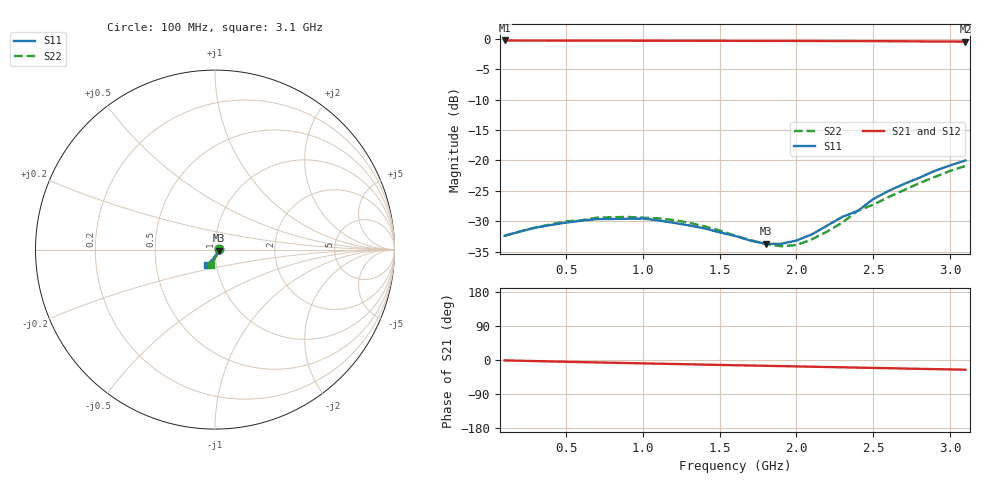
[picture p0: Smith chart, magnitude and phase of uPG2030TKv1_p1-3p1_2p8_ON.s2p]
! NEC Compound Semiconductor Devices Ltd.
! 21.January 2005
! uPG2030TK
! GaAs MMIC (0.1 - 3.1GHz SPDT switch)
! Vcont1=0v Vcont2=2.8v / IN-OUT1 ( ON )
! OUT2:50ohm termination
#  GHz  S  MA  R  50
!  f  S11  S21  S12  S22
!  GHz  MAG  ANG  MAG  ANG  MAG  ANG  MAG  ANG
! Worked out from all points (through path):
!   31 points, 100 MHz to 3.1 GHz, reference 50 ohm
!   highest |S21| = -0.25 dB at 100 MHz (marker M1); lowest = -0.4 dB at 3.1 GHz (marker M2)
!   group delay of S21, straight-line fit = 22.5 ps
!   lowest |S11| = -33.7 dB at 1.8 GHz (marker M3), VSWR 1.04, Z = 52 - j0.641 ohm
!   |S11| at or under -10 dB: start of sweep to end of sweep
!   |S22| runs from -34.1 to -20.9 dB; largest |S21 - S12| = 0.0034
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0.1  0.024 9.5  0.972 -1.0  0.971 -1.0  0.024 10.0
0.3  0.028 22.2  0.97 -2.9  0.97 -2.9  0.028 23.0
0.5  0.0308 28.7  0.969 -4.7  0.969 -4.7  0.0315 29.8
0.6  0.0319 32.3  0.9682 -5.6  0.9691 -5.6  0.0322 32.3
0.7  0.0329 32.0  0.9683 -6.4  0.9681 -6.4  0.0338 32.8
0.8  0.033 32.1  0.9677 -7.2  0.9676 -7.2  0.0341 33.7
1  0.0333 31.9  0.9672 -8.9  0.9665 -8.9  0.0338 34.4
1.1  0.0321 29.9  0.9666 -9.7  0.9667 -9.7  0.0334 32.8
1.3  0.0292 24.2  0.966 -11.3  0.9663 -11.3  0.0307 28.5
1.5  0.0256 14.9  0.9654 -13.0  0.9654 -13.0  0.0265 20.8
1.6  0.0239 7.1  0.9648 -13.8  0.965 -13.8  0.0241 14.3
1.7  0.0219 -4.1  0.9646 -14.5  0.9649 -14.5  0.0221 5.5
1.8  0.0206 -17.4  0.9642 -15.3  0.9644 -15.4  0.0205 -6.6
1.9  0.0206 -32.6  0.9635 -16.1  0.9638 -16.2  0.0197 -21.0
2  0.0219 -48.3  0.9631 -16.9  0.9631 -16.9  0.0201 -36.8
2.1  0.0246 -62.9  0.9622 -17.7  0.9623 -17.7  0.0224 -51.9
2.3  0.0344 -85.4  0.961 -19.3  0.9612 -19.3  0.0309 -74.1
2.4  0.0385 -93.2  0.9599 -20.1  0.9605 -20.1  0.0386 -79.6
2.5  0.0481 -98.2  0.9592 -20.9  0.9593 -20.9  0.0432 -86.6
2.6  0.0561 -103.5  0.9584 -21.6  0.958 -21.7  0.05 -91.0
2.9  0.082 -113.0  0.953 -24.1  0.956 -24.0  0.073 -100.0
3.1  0.1 -117.7  0.951 -25.6  0.952 -25.7  0.09 -104.5
